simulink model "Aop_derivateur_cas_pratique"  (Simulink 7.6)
settings: Solver=ode15s  StartTime=0.0  StopTime=3  RelTol=1e-3
libraries: fl_lib x10, nesl_utility x3, simulink x1

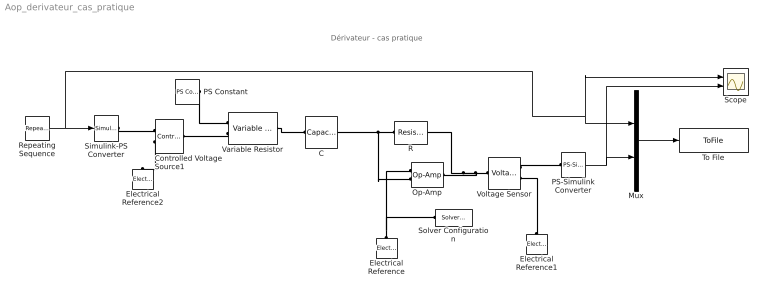
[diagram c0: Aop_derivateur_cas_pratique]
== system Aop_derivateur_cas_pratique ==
  note: Dérivateur - cas pratique
  C : fl_lib/Electrical/Electrical Elements/Capacitor  DialogController=NetworkEngine.DynNeDlgSource  SystemSampleTime=-1  c=100e-9 F  v0=0 V  r=1e-6 Ohm  g=0 1/Ohm  i_Log=off  v_Log=off  vc_Log=off  LocalVarNames=|current|voltage|power  LocalVarDescs=|Capacitor current (A)|Voltage across capacitor (V)|Power (W)  LocalVarLogging=[0 0 0]
  Controlled Voltage Source1 : fl_lib/Electrical/Electrical Sources/Controlled Voltage Source  DialogController=NetworkEngine.DynNeDlgSource  SystemSampleTime=-1  i_Log=off  v_Log=off  LocalVarNames=|current|voltage|power  LocalVarDescs=|Current (A)|Voltage (V)|Power (W)  LocalVarLogging=[0 0 0]
  Electrical Reference : fl_lib/Electrical/Electrical Elements/Electrical Reference  DialogController=NetworkEngine.DynNeDlgSource  SystemSampleTime=-1  i_Log=off  LocalVarNames=|i  LocalVarDescs=|i  LocalVarLogging=[]
  Electrical Reference1 : fl_lib/Electrical/Electrical Elements/Electrical Reference  DialogController=NetworkEngine.DynNeDlgSource  SystemSampleTime=-1  i_Log=off  LocalVarNames=|i  LocalVarDescs=|i  LocalVarLogging=[]
  Electrical Reference2 : fl_lib/Electrical/Electrical Elements/Electrical Reference  DialogController=NetworkEngine.DynNeDlgSource  SystemSampleTime=-1  i_Log=off  LocalVarNames=|i  LocalVarDescs=|i  LocalVarLogging=[]
  Mux : Mux  Inputs=2
  Op-Amp : fl_lib/Electrical/Electrical Elements/Op-Amp  DialogController=NetworkEngine.DynNeDlgSource  SystemSampleTime=-1  i1_Log=off  v1_Log=off  outI_Log=off  LocalVarNames=|i1|v1|outI  LocalVarDescs=|i1|v1|outI  LocalVarLogging=[]
  PS Constant : fl_lib/Physical Signals/Sources/PS Constant  DialogController=NetworkEngine.DynNeDlgSource  SystemSampleTime=-1  constant=100000  LocalVarLogging=[]
  PS-Simulink Converter : nesl_utility/PS-Simulink Converter  DialogController=NetworkEngine.DynNeUtilDlgSource  SystemSampleTime=-1  PhysicalDomain=network_engine_domain  LeftPortType=input  RightPortType=output  SubClassName=ps_output  Unit=1  AffineConversion=off
  R : fl_lib/Electrical/Electrical Elements/Resistor  DialogController=NetworkEngine.DynNeDlgSource  SystemSampleTime=-1  R=10e3 Ohm  i_Log=off  v_Log=off  LocalVarNames=|current|voltage|power  LocalVarDescs=|Resistor current (A)|Voltage across resistor (V)|Power (W)  LocalVarLogging=[0 0 0]
  Repeating Sequence : simulink/Sources/Repeating Sequence  SystemSampleTime=-1  rep_seq_t="[0  0.7 1.4 2.1 2.8 3.5 4.2 4.9]"  rep_seq_y="[0  0.1  0 .1 0  0.1  0 .1]"
  Scope : Scope  NumInputPorts=2
  Simulink-PS Converter : nesl_utility/Simulink-PS Converter  DialogController=NetworkEngine.DynNeUtilDlgSource  SystemSampleTime=-1  PhysicalDomain=network_engine_domain  LeftPortType=input  RightPortType=output  SubClassName=ps_input  Unit=1  AffineConversion=off  InputFilterTimeConstant=.001  UdotUserProvided=0
  Solver Configuration : nesl_utility/Solver Configuration  DialogController=NetworkEngine.DynNeUtilDlgSource  SystemSampleTime=-1  PhysicalDomain=network_engine_domain  LeftPortType=input  RightPortType=generic  SubClassName=solver  Accelerate=off  Profile=off  ResidualTolerance=1e-9  MaxNonlinIter=12  MaxModeIter=2  DoFixedCost=off  UseLocalSampling=off  DoDC=off  LinearAlgebra=Sparse  LocalSolverSampleTime=.001  LocalSolverChoice=NE_BACKWARD_EULER_ADVANCER  UseLocalSolver=off
  To File : ToFile  Filename=es.mat  MatrixName=xy
  Variable Resistor : fl_lib/Electrical/Electrical Elements/Variable Resistor  DialogController=NetworkEngine.DynNeDlgSource  SystemSampleTime=-1  Rmin=0 Ohm  i_Log=off  v_Log=off  LocalVarNames=|i|v  LocalVarDescs=|i|v  LocalVarLogging=[0 0]
  Voltage Sensor : fl_lib/Electrical/Electrical Sensors/Voltage Sensor  DialogController=NetworkEngine.DynNeDlgSource  SystemSampleTime=-1  i1_Log=off  v1_Log=off  LocalVarNames=|i1|v1  LocalVarDescs=|i1|v1  LocalVarLogging=[]
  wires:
  PS-Simulink Converter/1 -> Mux/2, Scope/2
  Mux/1 -> To File/1
  Repeating Sequence/1 -> Simulink-PS Converter/1, Mux/1, Scope/1
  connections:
  Electrical Reference/LConn1 -- Op-Amp/LConn1 -- Solver Configuration/RConn1
  R/LConn1 -- Op-Amp/LConn2 -- C/RConn1
  Voltage Sensor/LConn1 -- R/RConn1 -- Op-Amp/RConn1
  Electrical Reference1/LConn1 -- Voltage Sensor/RConn2
  Voltage Sensor/RConn1 -- PS-Simulink Converter/LConn1
  Controlled Voltage Source1/RConn2 -- Electrical Reference2/LConn1
  Simulink-PS Converter/RConn1 -- Controlled Voltage Source1/RConn1
  Variable Resistor/LConn2 -- Controlled Voltage Source1/LConn1
  Variable Resistor/RConn1 -- C/LConn1
  PS Constant/RConn1 -- Variable Resistor/LConn1
